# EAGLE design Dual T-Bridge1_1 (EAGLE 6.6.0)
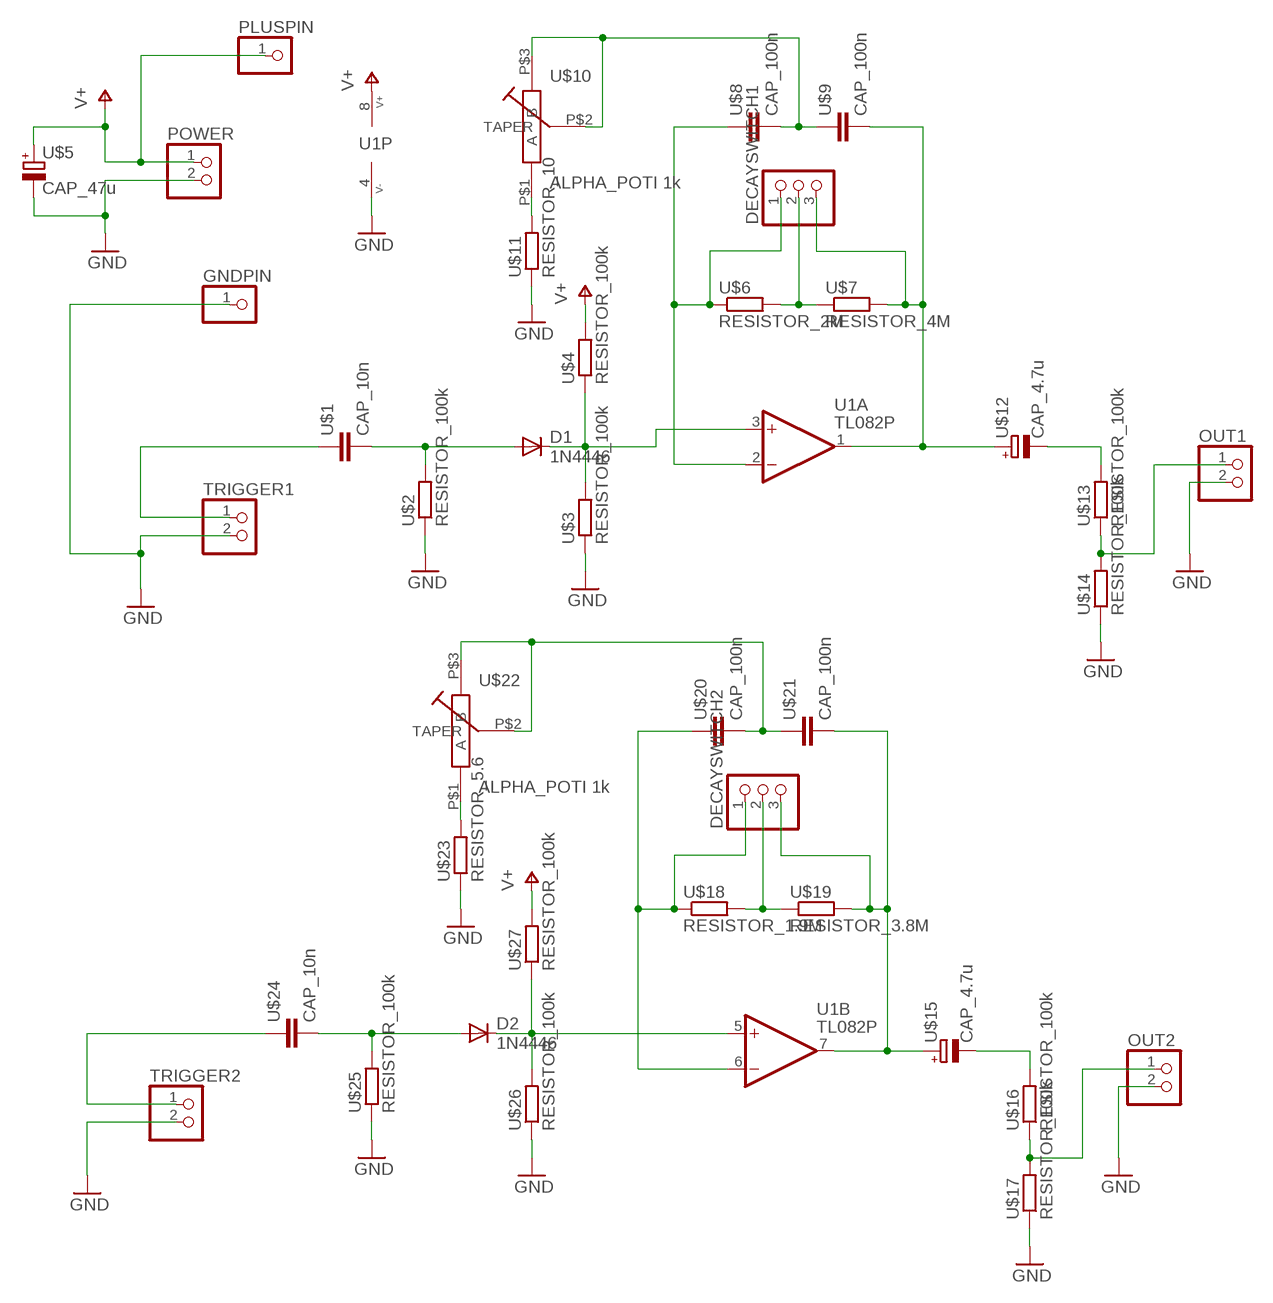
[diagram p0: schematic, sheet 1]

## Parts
D1  1N4446  [DO35-10]
D2  1N4446  [DO35-10]
DECAYSWITCH1  PINHD-1X3  [1X03]
DECAYSWITCH2  PINHD-1X3  [1X03]
GNDPIN  PINHD-1X1  [1X01]
OUT1  PINHD-1X2  [1X02]
OUT2  PINHD-1X2  [1X02]
PLUSPIN  PINHD-1X1  [1X01]
POWER  PINHD-1X2  [1X02]
TRIGGER1  PINHD-1X2  [1X02]
TRIGGER2  PINHD-1X2  [1X02]
U1  TL082P  [DIL08]
U$1  CAP_10n  CAP_NONPOL  [CAP_NONPOL]
U$2  RESISTOR_100k  RESISTOR_10MM  [RESISTOR_10MM]
U$3  RESISTOR_100k  RESISTOR_10MM  [RESISTOR_10MM]
U$4  RESISTOR_100k  RESISTOR_10MM  [RESISTOR_10MM]
U$5  CAP_47u  CAP_POL  [CAP_POL]
U$6  RESISTOR_2M  RESISTOR_10MM  [RESISTOR_10MM]
U$7  RESISTOR_4M  RESISTOR_10MM  [RESISTOR_10MM]
U$8  CAP_100n  CAP_NONPOL  [CAP_NONPOL]
U$9  CAP_100n  CAP_NONPOL  [CAP_NONPOL]
U$10  ALPHA_POTI 1k  ALPHA_POTI  [ALPHA_PRINT]
U$11  RESISTOR_10  RESISTOR_10MM  [RESISTOR_10MM]
U$12  CAP_4.7u  CAP_POL  [CAP_POL]
U$13  RESISTOR_100k  RESISTOR_10MM  [RESISTOR_10MM]
U$14  RESISTOR_100k  RESISTOR_10MM  [RESISTOR_10MM]
U$15  CAP_4.7u  CAP_POL  [CAP_POL]
U$16  RESISTOR_100k  RESISTOR_10MM  [RESISTOR_10MM]
U$17  RESISTOR_100k  RESISTOR_10MM  [RESISTOR_10MM]
U$18  RESISTOR_1.9M  RESISTOR_10MM  [RESISTOR_10MM]
U$19  RESISTOR_3.8M  RESISTOR_10MM  [RESISTOR_10MM]
U$20  CAP_100n  CAP_NONPOL  [CAP_NONPOL]
U$21  CAP_100n  CAP_NONPOL  [CAP_NONPOL]
U$22  ALPHA_POTI 1k  ALPHA_POTI  [ALPHA_PRINT]
U$23  RESISTOR_5.6  RESISTOR_10MM  [RESISTOR_10MM]
U$24  CAP_10n  CAP_NONPOL  [CAP_NONPOL]
U$25  RESISTOR_100k  RESISTOR_10MM  [RESISTOR_10MM]
U$26  RESISTOR_100k  RESISTOR_10MM  [RESISTOR_10MM]
U$27  RESISTOR_100k  RESISTOR_10MM  [RESISTOR_10MM]

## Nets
GND: GNDPIN.1 OUT1.2 OUT2.2 POWER.2 TRIGGER1.2 TRIGGER2.2 U1.4(P:V-) U$2.1 U$3.1 U$5.- U$11.1 U$14.1 U$17.1 U$23.1 U$25.1 U$26.1
N$1: TRIGGER1.1 U$1.1
N$2: D1.A U$1.2 U$2.2
N$3: D1.C U1.3(A:+IN) U$3.2 U$4.1
N$4: U$20.2 U$21.1 U$22.P$2(TAPER) U$22.P$3(B)
N$5: OUT2.1 U$16.1 U$17.2
N$6: U$15.- U$16.2
N$7: DECAYSWITCH1.1 U1.2(A:-IN) U$6.1 U$8.1
N$8: DECAYSWITCH1.2 U$6.2 U$7.1
N$9: DECAYSWITCH1.3 U1.1(A:OUT) U$7.2 U$9.2 U$12.+
N$10: DECAYSWITCH2.1 U1.6(B:-IN) U$18.1 U$20.1
N$11: DECAYSWITCH2.2 U$18.2 U$19.1
N$12: U$8.2 U$9.1 U$10.P$2(TAPER) U$10.P$3(B)
N$13: DECAYSWITCH2.3 U1.7(B:OUT) U$15.+ U$19.2 U$21.2
N$14: U$10.P$1(A) U$11.2
N$16: OUT1.1 U$13.1 U$14.2
N$17: U$12.- U$13.2
N$18: U$22.P$1(A) U$23.2
N$19: TRIGGER2.1 U$24.1
N$20: D2.A U$24.2 U$25.2
N$21: D2.C U1.5(B:+IN) U$26.2 U$27.1
V+: PLUSPIN.1 POWER.1 U1.8(P:V+) U$4.2 U$5.+ U$27.2

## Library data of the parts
D1 D2 = diode:1N4446: DIODE
DECAYSWITCH1 DECAYSWITCH2 = pinhead:PINHD-1X3: PIN HEADER
GNDPIN PLUSPIN = pinhead:PINHD-1X1: PIN HEADER
OUT1 OUT2 POWER TRIGGER1 TRIGGER2 = pinhead:PINHD-1X2: PIN HEADER
U1 = op-amp:TL082: JFET OP-AMP - Dual
U$1 U$8 U$9 U$20 U$21 U$24 = eigene:CAP_NONPOL
U$2-U$4 U$6 U$7 U$11 U$13 U$14 U$16-U$19 U$23 U$25-U$27 = eigene:RESISTOR_10MM
U$5 U$12 U$15 = eigene:CAP_POL
U$10 U$22 = eigene:ALPHA_POTI

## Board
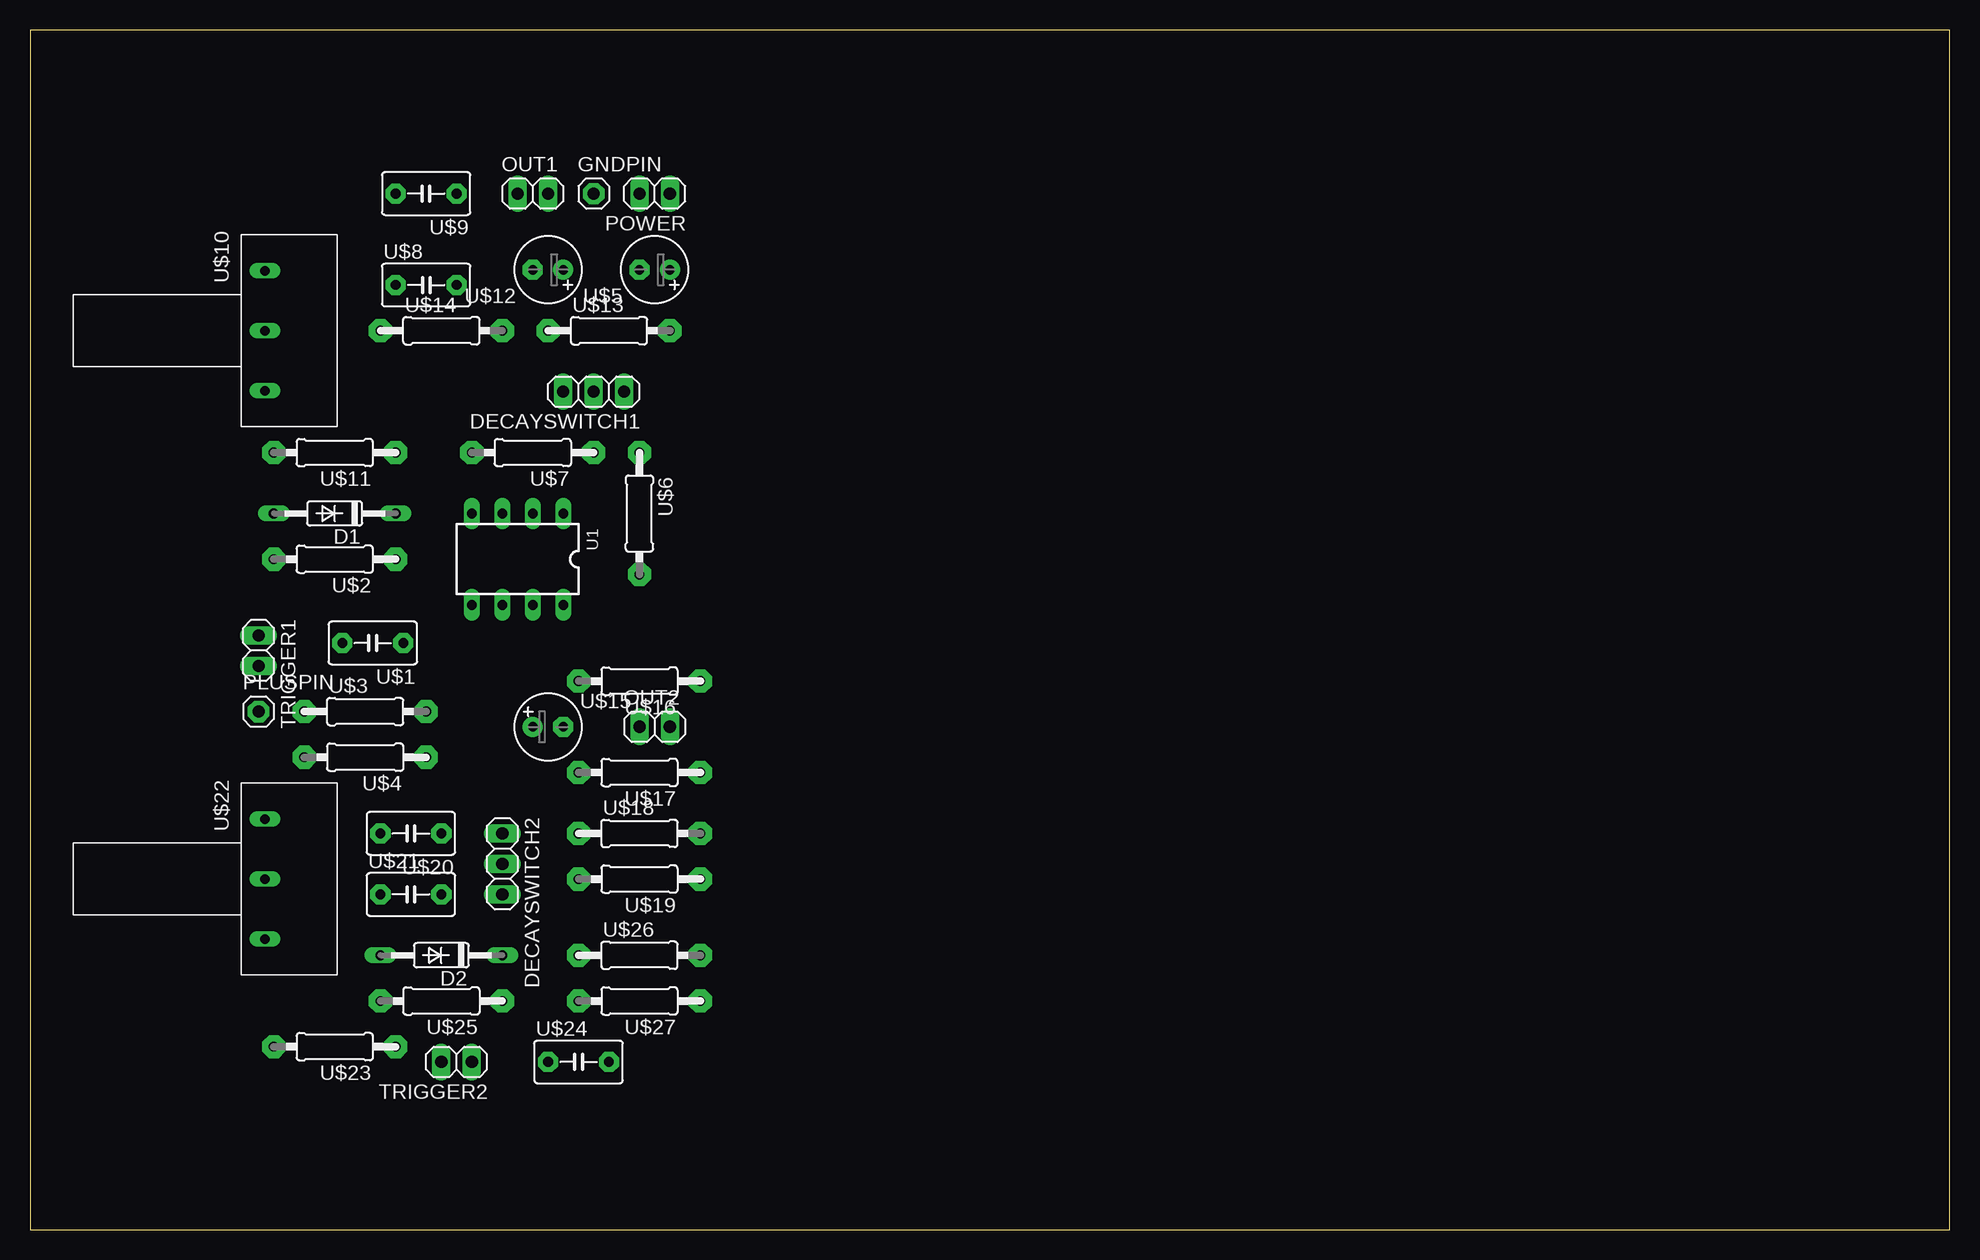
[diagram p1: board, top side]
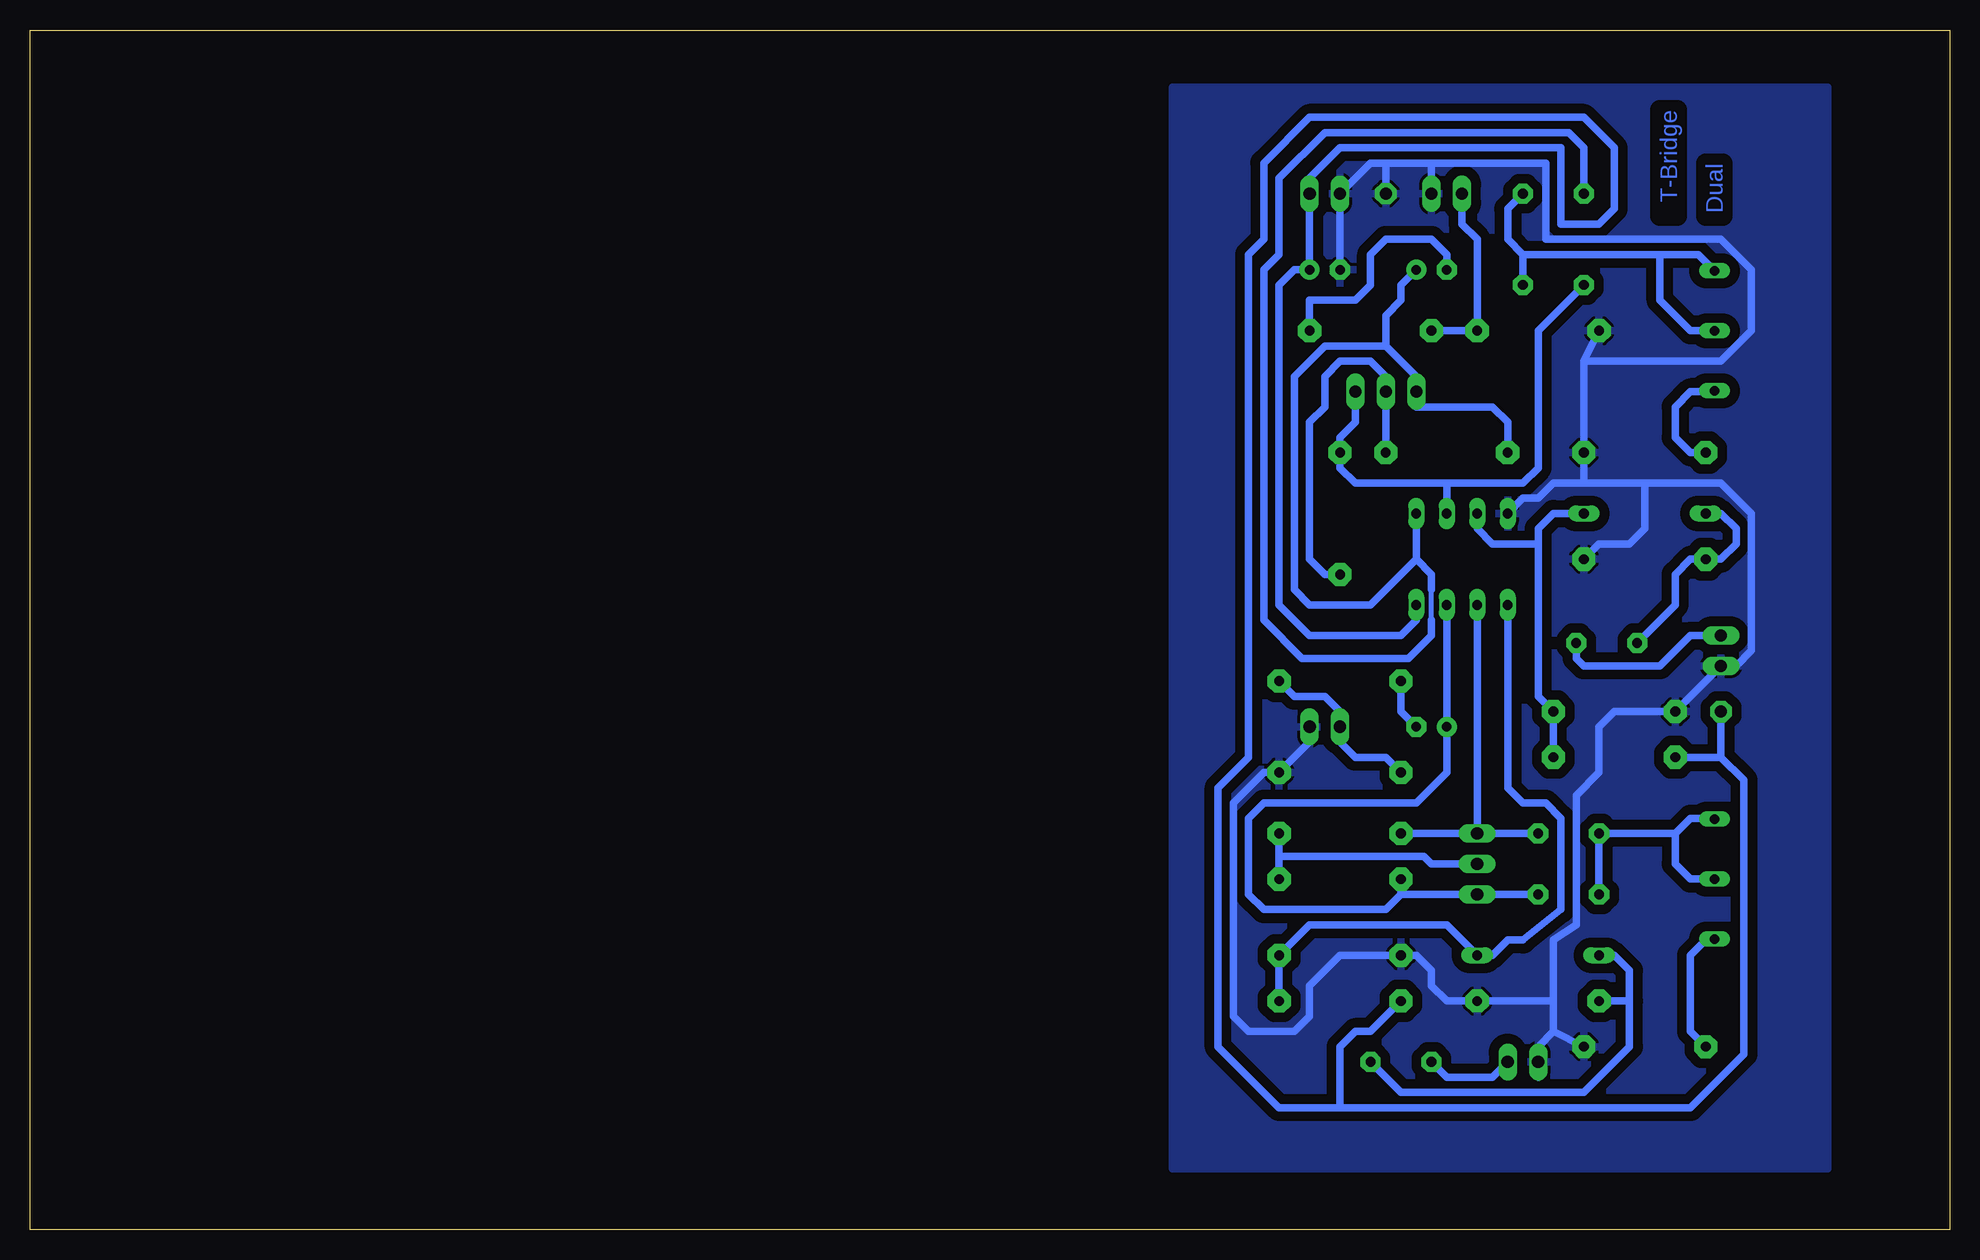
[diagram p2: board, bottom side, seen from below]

Size 160 x 100 mm. Coordinates in mm from the lower left corner, seen from the top.
Outline: 0,0 160,0 160,100 0,100 0,0
Copper layers (1*16): Top 0.035mm / dielectric 1.5mm / Bottom 0.035mm
Design rules "default": minimum track width 10mil, minimum drill 24mil, track to track 8mil, track to pad 8mil, pad to pad 8mil, via to via 8mil, smd to smd 8mil, copper to edge 40mil, drill to drill 8mil, minimum pad ring 10mil, minimum via ring 8mil, stop-mask expansion 4mil, vias tented up to drill 0mil, thermal gap 10mil

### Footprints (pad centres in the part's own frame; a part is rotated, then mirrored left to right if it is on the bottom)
DO35-10 = drill 0.813 long: A 5.08,0; C -5.08,0
1X03 = drill 1.016 long: 1 -2.54,0; 2 0,0; 3 2.54,0
1X01 = drill 1.016 pad 1.778 octagon: 1 0,0
1X02 = drill 1.016 long: 1 -1.27,0; 2 1.27,0
DIL08 = drill 0.813 long: 1 -3.81,-3.81; 2 -1.27,-3.81; 3 1.27,-3.81; 4 3.81,-3.81; 5 3.81,3.81; 6 1.27,3.81; 7 -1.27,3.81; 8 -3.81,3.81
CAP_NONPOL = drill 0.813 pad 1.676 octagon: 1 -2.54,0; 2 2.54,0
RESISTOR_10MM = drill 0.813 pad 1.93 octagon: 1 -5.08,0; 2 5.08,0
CAP_POL = drill 0.813 pad 1.676: + -1.27,0 | drill 0.813 pad 1.676 octagon: - 1.27,0
ALPHA_PRINT = drill 0.8 long: P$1 -5,2; P$2 0,2; P$3 5,2

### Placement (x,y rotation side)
D1  25.4,59.69 180 top
D2  34.29,22.86 180 top
DECAYSWITCH1  46.99,69.85 180 top
DECAYSWITCH2  39.37,30.48 270 top
GNDPIN  46.99,86.36 0 top
OUT1  41.91,86.36 0 top
OUT2  52.07,41.91 0 top
PLUSPIN  19.05,43.18 0 top
POWER  52.07,86.36 180 top
TRIGGER1  19.05,48.26 270 top
TRIGGER2  35.56,13.97 180 top
U1  40.64,55.88 180 top
U$1  28.57,48.9 180 top
U$2  25.4,55.88 180 top
U$3  27.94,43.18 0 top
U$4  27.94,39.37 180 top
U$5  52.07,80.01 180 top
U$6  50.8,59.69 270 top
U$7  41.91,64.77 180 top
U$8  33.02,78.74 0 top
U$9  33.02,86.36 180 top
U$10  21.59,74.93 90 top
U$11  25.4,64.77 180 top
U$12  43.18,80.01 180 top
U$13  48.26,74.93 0 top
U$14  34.29,74.93 0 top
U$15  43.18,41.91 0 top
U$16  50.8,45.72 180 top
U$17  50.8,38.1 180 top
U$18  50.8,33.02 0 top
U$19  50.8,29.21 180 top
U$20  31.75,33.02 180 top
U$21  31.75,27.94 0 top
U$22  21.59,29.21 90 top
U$23  25.4,15.24 180 top
U$24  45.72,13.97 0 top
U$25  34.29,19.05 180 top
U$26  50.8,22.86 0 top
U$27  50.8,19.05 180 top

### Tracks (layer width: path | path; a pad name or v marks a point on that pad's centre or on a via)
GND
  Bottom 0.61: U$14.1 30.48,72.39 | 30.48,72.39 U$11.1 30.48,62.23 | U$5.- POWER.2 48.26,88.9 46.99,88.9 | 46.99,88.9 43.18,88.9 | 43.18,88.9 33.66,88.9 33.66,82.55 19.05,82.55 16.51,80.01 16.51,74.93 19.05,72.39 30.48,72.39 | U1.4 35.56,60.96 34.29,60.96 33.02,62.23 30.48,62.23 | U$23.1 33.02,16.51 | 33.02,16.51 33.02,19.05 | 33.02,19.05 33.02,24.13 31.11,25.4 31.11,36.2 29.21,38.1 29.21,41.91 27.94,43.18 U$3.1 TRIGGER1.2 17.78,46.99 16.51,48.26 16.51,59.69 19.05,62.23 25.4,62.23 | 34.29,12.7 TRIGGER2.2 34.29,15.24 33.02,16.51 | U$2.1 29.21,57.15 26.67,57.15 25.4,58.42 25.4,62.23 | 30.48,62.23 25.4,62.23 | OUT1.2 43.18,88.9 | OUT2.2 53.34,40.64 U$17.1 57.15,38.1 59.69,35.56 59.69,17.78 58.42,16.51 54.61,16.51 53.34,17.78 53.34,20.32 50.8,22.86 U$26.1 44.45,22.86 43.18,21.59 43.18,20.32 41.91,19.05 U$25.1 33.02,19.05 | GNDPIN.1 46.99,88.9
  pour Bottom (isolate 0.813): 10.16,95.25 64.77,95.25 64.77,5.08 10.16,5.08
N$1
  Bottom 0.61: TRIGGER1.1 21.59,49.53 24.13,46.99 30.48,46.99 31.11,47.62 U$1.1
N$2
  Bottom 0.61: D1.A 19.05,59.69 17.78,58.42 17.78,57.15 19.05,55.88 U$2.2 21.59,55.88 22.86,54.61 22.86,52.07 U$1.2
N$3
  Bottom 0.61: U1.3 39.37,58.42 38.1,57.15 34.29,57.15 | D1.C 33.02,59.69 34.29,58.42 34.29,57.15 | U$4.1 U$3.2 34.29,44.45 34.29,57.15
N$4
  Bottom 0.61: 22.86,33.02 22.86,30.48 21.59,29.21 U$22.P$2 | 22.86,33.02 U$20.2 U$21.1 | U$22.P$3 19.67,34.29 21.59,34.29 22.86,33.02
N$5
  Bottom 0.61: U$17.2 46.99,39.37 49.53,39.37 50.8,40.64 OUT2.1 50.8,43.18 52.07,44.45 54.61,44.45 U$16.1
N$6
  Bottom 0.61: U$15.- 45.72,43.18 U$16.2
N$7
  Bottom 0.61: DECAYSWITCH1.1 49.53,67.31 50.8,66.04 U$6.1 50.8,63.5 49.53,62.23 41.91,62.23 | 41.91,62.23 35.56,62.23 34.29,63.5 34.29,74.93 U$8.1 | U1.2 41.91,62.23
N$8
  Bottom 0.61: U$7.1 DECAYSWITCH1.2 46.99,71.12 48.26,72.39 50.8,72.39 52.07,71.12 52.07,68.58 53.34,67.31 53.34,55.88 52.07,54.61 U$6.2
N$9
  Bottom 0.406: 43.18,50.8 43.18,53.34
  Bottom 0.61: U$7.2 36.83,67.31 38.1,68.58 44.45,68.58 DECAYSWITCH1.3 44.45,71.12 46.99,73.66 | U$9.2 30.48,90.17 31.75,91.44 52.07,91.44 55.88,87.63 55.88,81.28 57.15,80.01 57.15,50.8 53.98,47.62 45.09,47.62 43.18,49.53 43.18,50.8 | 46.99,73.66 46.99,76.2 45.72,77.47 45.72,78.74 U$12.+ | 46.99,73.66 52.07,73.66 54.61,71.12 54.61,53.34 53.34,52.07 48.26,52.07 44.45,55.88 | U1.1 44.45,55.88 | 43.18,53.34 43.18,54.61 44.45,55.88
N$10
  Bottom 0.61: U1.6 DECAYSWITCH2.1 | U$20.1 DECAYSWITCH2.1 | DECAYSWITCH2.1 U$18.1
N$11
  Bottom 0.61: U$18.2 55.88,31.11 | 55.88,31.11 U$19.1 | 55.88,31.11 43.81,31.11 43.18,30.48 DECAYSWITCH2.2
N$12
  Bottom 0.61: U$10.P$3 20.94,81.28 24.13,81.28 | 24.13,81.28 35.56,81.28 | U$10.P$2 21.59,74.93 24.13,77.47 24.13,81.28 | U$9.1 36.83,85.09 36.83,82.55 35.56,81.28 | 35.56,81.28 U$8.2
N$13
  Bottom 0.61: U1.7 U$15.+ 41.91,38.1 44.45,35.56 57.15,35.56 58.42,34.29 58.42,27.94 57.15,26.67 46.99,26.67 45.72,27.94 | U$21.2 DECAYSWITCH2.3 45.72,27.94 | 45.72,27.94 U$19.2
N$14
  Bottom 0.61: U$10.P$1 19.67,69.85 21.59,69.85 22.86,68.58 22.86,66.04 21.59,64.77 U$11.2
N$16
  Bottom 0.61: U$13.1 U$14.2 39.37,82.55 40.64,83.82 OUT1.1
N$17
  Bottom 0.61: U$13.2 53.34,77.47 49.53,77.47 48.26,78.74 48.26,81.28 46.99,82.55 43.18,82.55 41.91,81.28 U$12.-
N$18
  Bottom 0.61: U$22.P$1 20.24,24.21 21.59,22.86 21.59,16.51 U$23.2
N$19
  Bottom 0.61: TRIGGER2.1 38.1,12.7 41.91,12.7 U$24.1
N$20
  Bottom 0.61: U$24.2 45.72,11.43 30.48,11.43 26.67,15.24 26.67,19.05 | 26.67,19.05 26.67,21.59 27.94,22.86 D2.A | U$25.2 26.67,19.05
N$21
  Bottom 0.61: U$27.1 U$26.2 53.34,25.4 41.91,25.4 D2.C 38.1,22.86 36.83,24.13 35.56,24.13 32.38,26.67 32.38,34.29 33.66,35.56 35.56,35.56 36.83,36.83 U1.5
V+
  Bottom 0.61: U1.8 44.45,50.8 45.72,49.53 53.34,49.53 55.88,52.07 55.88,78.74 54.61,80.01 U$5.+ POWER.1 53.34,87.63 50.8,90.17 32.38,90.17 32.38,83.82 29.21,83.82 27.94,85.09 27.94,90.17 30.48,92.71 53.34,92.71 57.15,88.9 57.15,82.55 58.42,81.28 58.42,39.37 60.96,36.83 60.96,15.24 55.88,10.16 50.8,10.16 | U$4.2 19.05,39.37 | 50.8,10.16 21.59,10.16 17.14,14.61 17.14,37.47 19.05,39.37 | U$27.2 48.26,16.51 49.53,16.51 50.8,15.24 50.8,10.16 | PLUSPIN.1 19.05,39.37

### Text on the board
Bottom: T-Bridge | Dual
